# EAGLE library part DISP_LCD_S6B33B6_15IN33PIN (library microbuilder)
1.5" 128x128 Pixel 65K CSTN LCD with S6B33B6 Controller 33-Pins
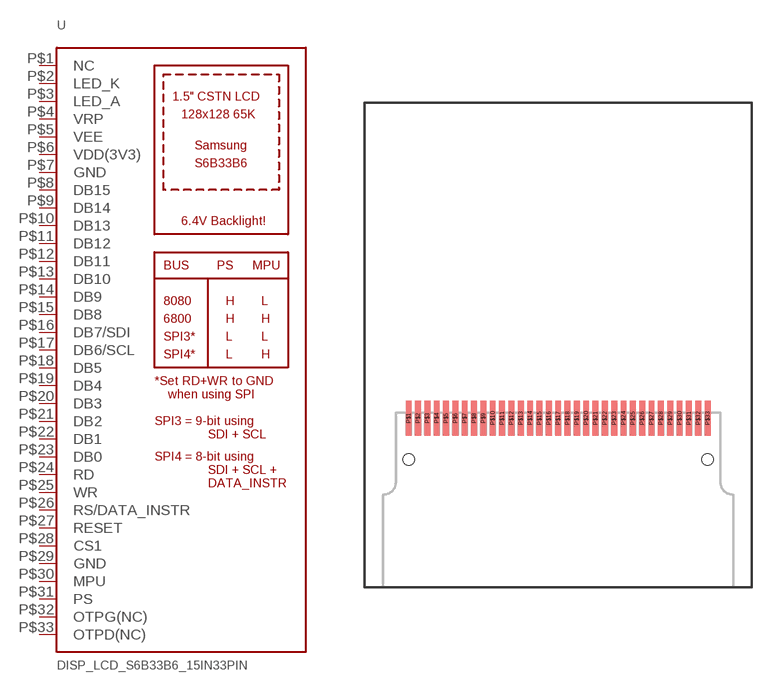
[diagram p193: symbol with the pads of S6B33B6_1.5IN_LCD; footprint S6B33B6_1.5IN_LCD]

Designator prefix U

## DISP_LCD_S6B33B6_15IN33PIN  [S6B33B6_1.5IN_LCD]
P$1  NC  nc
P$2  LED_K
P$3  LED_A
P$4  VRP  out
P$5  VEE  in
P$6  VDD(3V3)  pwr
P$7  GND  pwr
P$8  DB15
P$9  DB14
P$10  DB13
P$11  DB12
P$12  DB11
P$13  DB10
P$14  DB9
P$15  DB8
P$16  DB7/SDI
P$17  DB6/SCL
P$18  DB5
P$19  DB4
P$20  DB3
P$21  DB2
P$22  DB1
P$23  DB0
P$24  RD  in
P$25  WR  in
P$26  RS/DATA_INSTR  in
P$27  RESET  in
P$28  CS1  in
P$29  GND  pwr
P$30  MPU  in
P$31  PS  in
P$32  OTPG(NC)  nc
P$33  OTPD(NC)  nc

## Footprint S6B33B6_1.5IN_LCD (pad centres in mm)
Mystery 1.5" S6B33B6X TFT LCD BAsed on manual measurements with a caliper since no mechanical diagram was available, but should be relatively close.
smd 0.5 x 3: P$1 -12.8,-6.25; P$2 -12,-6.25; P$3 -11.2,-6.25; P$4 -10.4,-6.25; P$5 -9.6,-6.25; P$6 -8.8,-6.25; P$7 -8,-6.25; P$8 -7.2,-6.25; P$9 -6.4,-6.25; P$10 -5.6,-6.25; P$11 -4.8,-6.25; P$12 -4,-6.25; P$13 -3.2,-6.25; P$14 -2.4,-6.25; P$15 -1.6,-6.25; P$16 -0.8,-6.25; P$17 0,-6.25; P$18 0.8,-6.25; P$19 1.6,-6.25; P$20 2.4,-6.25; P$21 3.2,-6.25; P$22 4,-6.25; P$23 4.8,-6.25; P$24 5.6,-6.25; P$25 6.4,-6.25; P$26 7.2,-6.25; P$27 8,-6.25; P$28 8.8,-6.25; P$29 9.6,-6.25; P$30 10.4,-6.25; P$31 11.2,-6.25; P$32 12,-6.25; P$33 12.8,-6.25
hole 1 at 12.8,-9.8
hole 1 at -12.8,-9.8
